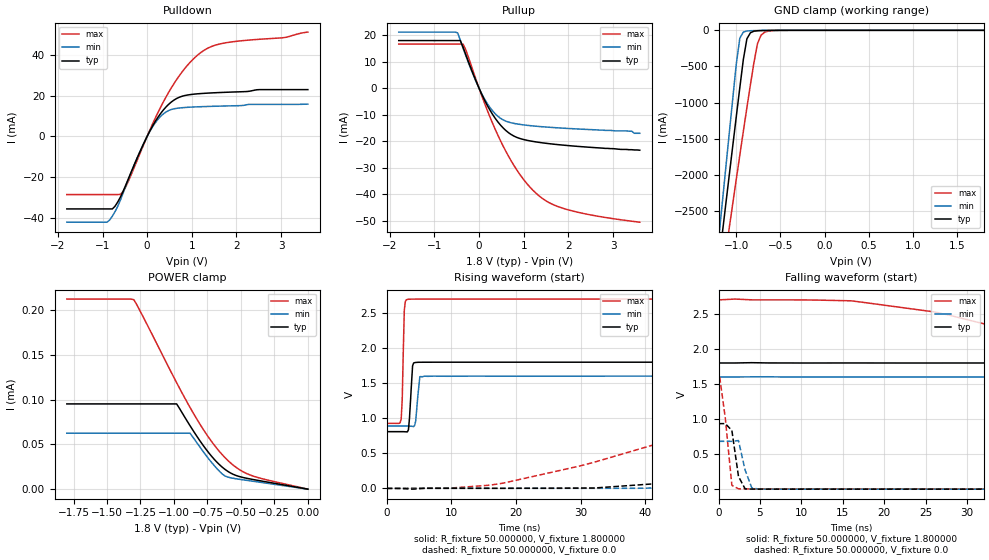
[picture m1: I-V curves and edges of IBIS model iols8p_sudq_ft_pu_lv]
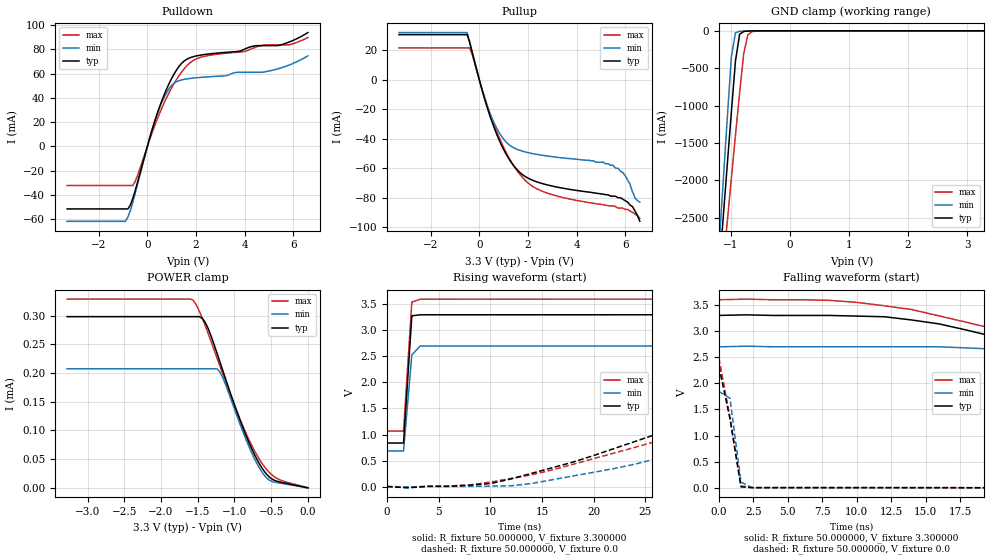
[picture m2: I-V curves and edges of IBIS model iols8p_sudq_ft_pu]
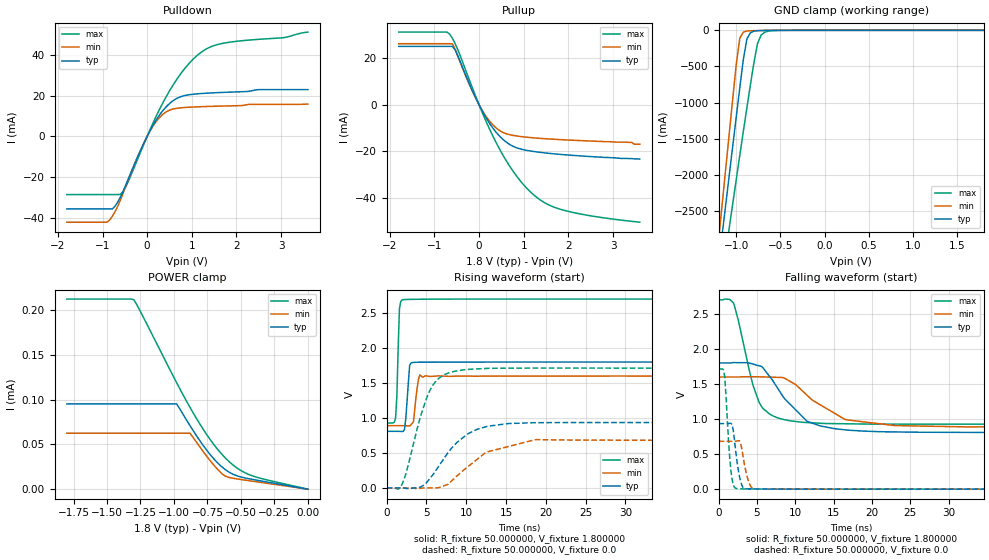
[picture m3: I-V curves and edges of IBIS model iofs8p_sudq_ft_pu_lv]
| IBIS file stm32wl33_vfqfpn32.ibs
[IBIS ver] 4.2
[File name] stm32wl33_vfqfpn32.ibs
[File Rev] 1.0
[Date]  24-06-2024
[Source] Data Created at STMicroelectronics
[Notes]  File originated from ELDO simulations.
[Disclaimer]  This information is for modeling purpose only and is
   not guaranteed. The information is subject to change without
   notice.
[Copyright] Copyright 2024 STMicroelectronics Inc.
|   Component stm32wl33_vfqfpn32
[Component] stm32wl33_vfqfpn32
[Manufacturer] STMicroelectronics
[Package]
| variable   typ   min   max
R_pkg  0  NA  NA
L_pkg  0  NA  NA
C_pkg  0  NA  NA
[Pin]   signal_name   model_name
1  PA2  io8prog2m25m50m120m_sudq_ft
2  PA3  io8prog2m25m50m120m_sudq_ft
3  VDD_1  power
4  PA0  io8prog2m25m50m120m_sudq_i2c_ft
5  PA11  io8prog2m25m50m120m_sudq_ft
6  PA10  io8prog2m25m50m120m_sudq_ft
7  PA9  io8prog2m25m50m120m_sudq_ft
8  PA8  io8prog2m25m50m120m_sudq_ft
9  PB6  io8prog2m25m50m120m_sudq_i2c_ft
10  PB12  io8prog2m25m50m120m_sudq_ft
11  PB13  io8prog2m25m50m120m_sudq_ft
12  PB14  io8prog2m25m50m120m_sudq_ft
13  PB15  io8prog2m25m50m120m_sudq_ft
14  LPAWUR  nc
15  RX  nc
16  EXTGND  gnd
17  TX_HP  nc
18  TX  nc
19  VDDRF  nc
20  OSCOUT  nc
21  OSCIN  nc
22  PA1  io8prog2m25m50m120m_sudq_i2c_ft
23  PB7  io8prog2m25m50m120m_sudq_i2c_ft
24  NRST  nc
25  VDDSD  nc
26  VLXSD  nc
27  VSSSD  nc
28  VFBSD  nc
29  VCAP  nc
30  PB0  io8prog2m25m50m120m_sudq_ft
31  PB1  io8prog2m25m50m120m_sudq_ft
32  PB2  io8prog2m25m50m120m_sudq_ft
0  EXTGND  gnd
[Package Model]   4l0-qfn-5x5-32-100mhz-230713
[Pin Mapping]   pulldown_ref   pullup_ref   | Comment
1  gndio  vddio
2  gndio  vddio
3  nc  vddio
4  gndio  vddio
5  gndio  vddio
6  gndio  vddio
7  gndio  vddio
8  gndio  vddio
9  gndio  vddio
10  gndio  vddio
11  gndio  vddio
12  gndio  vddio
13  gndio  vddio
14  nc  nc
15  nc  nc
16  gndio  nc
17  nc  nc
18  nc  nc
19  nc  nc
20  nc  nc
21  nc  nc
22  gndio  vddio
23  gndio  vddio
24  nc  nc
25  nc  nc
26  nc  nc
27  nc  nc
28  nc  nc
29  nc  nc
30  gndio  vddio
31  gndio  vddio
32  gndio  vddio
0  gndio  nc
[Model Selector] io8prog2m25m50m120m_sudq_ft
iols8p_sudq_ft_pd_lv  "IO low speed, PD=40kOhm - 1P8V"
iols8p_sudq_ft_pu_lv  "IO low speed, PU=40kOhm - 1P8V"
iols8p_sudq_ft_lv  "IO low speed - 1P8V"
iols8p_sudq_ft_pd  "IO low speed, PD=40kOhm - 3P3V"
iols8p_sudq_ft_pu  "IO low speed, PU=40kOhm - 3P3V"
iols8p_sudq_ft  "IO low speed - 3P3V"
iofs8p_sudq_ft_pd_lv  "IO full speed, PD=40kOhm - 1P8V"
iofs8p_sudq_ft_pu_lv  "IO full speed, PU=40kOhm - 1P8V"
iofs8p_sudq_ft_lv  "IO full speed - 1P8V"
iofs8p_sudq_ft_pd  "IO full speed, PD=40kOhm - 3P3V"
iofs8p_sudq_ft_pu  "IO full speed, PU=40kOhm - 3P3V"
iofs8p_sudq_ft  "IO full speed - 3P3V"
ioms8p_sudq_ft_pd_lv  "IO medium speed, PD=40kOhm - 1P8V"
ioms8p_sudq_ft_pu_lv  "IO medium speed, PU=40kOhm - 1P8V"
ioms8p_sudq_ft_lv  "IO medium speed - 1P8V"
ioms8p_sudq_ft_pd  "IO medium speed, PD=40kOhm - 3P3V"
ioms8p_sudq_ft_pu  "IO medium speed, PU=40kOhm - 3P3V"
ioms8p_sudq_ft  "IO medium speed - 3P3V"
iohs8p_sudq_ft_pd_lv  "IO high speed, PD=40kOhm - 1P8V"
iohs8p_sudq_ft_pu_lv  "IO high speed, PU=40kOhm - 1P8V"
iohs8p_sudq_ft_lv  "IO high speed - 1P8V"
iohs8p_sudq_ft_pd  "IO high speed, PD=40kOhm - 3P3V"
iohs8p_sudq_ft_pu  "IO high speed, PU=40kOhm - 3P3V"
iohs8p_sudq_ft  "IO high speed - 3P3V"
[Model Selector] io8prog2m25m50m120m_sudq_i2c_ft
iols8p_sudq_ft_pd_lv  "IO low speed, PD=40kOhm - 1P8V"
iols8p_sudq_ft_pu_lv  "IO low speed, PU=40kOhm - 1P8V"
iols8p_sudq_ft_lv  "IO low speed - 1P8V"
iols8p_sudq_ft_pd  "IO low speed, PD=40kOhm - 3P3V"
iols8p_sudq_ft_pu  "IO low speed, PU=40kOhm - 3P3V"
iols8p_sudq_ft  "IO low speed - 3P3V"
iofs8p_sudq_ft_pd_lv  "IO full speed, PD=40kOhm - 1P8V"
iofs8p_sudq_ft_pu_lv  "IO full speed, PU=40kOhm - 1P8V"
iofs8p_sudq_ft_lv  "IO full speed - 1P8V"
iofs8p_sudq_ft_pd  "IO full speed, PD=40kOhm - 3P3V"
iofs8p_sudq_ft_pu  "IO full speed, PU=40kOhm - 3P3V"
iofs8p_sudq_ft  "IO full speed - 3P3V"
ioms8p_sudq_ft_pd_lv  "IO medium speed, PD=40kOhm - 1P8V"
ioms8p_sudq_ft_pu_lv  "IO medium speed, PU=40kOhm - 1P8V"
ioms8p_sudq_ft_lv  "IO medium speed - 1P8V"
ioms8p_sudq_ft_pd  "IO medium speed, PD=40kOhm - 3P3V"
ioms8p_sudq_ft_pu  "IO medium speed, PU=40kOhm - 3P3V"
ioms8p_sudq_ft  "IO medium speed - 3P3V"
iohs8p_sudq_ft_pd_lv  "IO high speed, PD=40kOhm - 1P8V"
iohs8p_sudq_ft_pu_lv  "IO high speed, PU=40kOhm - 1P8V"
iohs8p_sudq_ft_lv  "IO high speed - 1P8V"
iohs8p_sudq_ft_pd  "IO high speed, PD=40kOhm - 3P3V"
iohs8p_sudq_ft_pu  "IO high speed, PU=40kOhm - 3P3V"
iohs8p_sudq_ft  "IO high speed - 3P3V"
io8_ft_i2c_ls_1v2   "GPIO I2C open-drain - 5V tolerant - 1.2V range - Low speed"
io8_ft_i2c_ms_1v2   "GPIO I2C open-drain - 5V tolerant - 1.2V range - Med speed"
io8_ft_i2c_fs_1v2   "GPIO I2C open-drain - 5V tolerant - 1.2V range - Fast speed"
io8_ft_i2c_hs_1v2   "GPIO I2C open-drain - 5V tolerant - 1.2V range - High speed"
io8_ft_i2c_ls_1v8   "GPIO I2C open-drain - 5V tolerant - 1.8V range - Low speed"
io8_ft_i2c_ms_1v8   "GPIO I2C open-drain - 5V tolerant - 1.8V range - Med speed"
io8_ft_i2c_fs_1v8   "GPIO I2C open-drain - 5V tolerant - 1.8V range - Fast speed"
io8_ft_i2c_hs_1v8   "GPIO I2C open-drain - 5V tolerant - 1.8V range - High speed"
io8_ft_i2c_ls_3v3   "GPIO I2C open-drain - 5V tolerant - 3.3V range - Low speed"
io8_ft_i2c_ms_3v3   "GPIO I2C open-drain - 5V tolerant - 3.3V range - Med speed"
io8_ft_i2c_fs_3v3   "GPIO I2C open-drain - 5V tolerant - 3.3V range - Fast speed"
io8_ft_i2c_hs_3v3   "GPIO I2C open-drain - 5V tolerant - 3.3V range - High speed"
io8_ft_i2c_fmp_3v3   "GPIO I2C open-drain fm+ - 5V tolerant - 3.3V range"
[Define Package Model]  4l0-qfn-5x5-32-100mhz-230713
[Manufacturer]  Unknown
[OEM]  Unknown
[Description]  None
[Number Of Pins]  32
[Pin Numbers]
| Pin Num   Terminal Name
14 | LPAWUR
4 | PA0
22 | PA1
1 | PA2
2 | PA3
8 | PA8
7 | PA9
6 | PA10
5 | PA11
30 | PB0
31 | PB1
32 | PB2
9 | PB6
23 | PB7
10 | PB12
11 | PB13
12 | PB14
13 | PB15
21 | OSCIN
20 | OSCOUT
27 | VSSSD
24 | NRST
15 | RX
28 | VFBSD
26 | VLXSD
18 | TX
17 | TX_HP
19 | VDDRF
3 | VDD_1
29 | VCAP
25 | VDDSD
16 | EXTGND
[Model Data]
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[End Model Data]
[End Package Model]
| Models and submodels in the file (37): iols8p_sudq_ft_pd_lv (I/O), iols8p_sudq_ft_pu_lv (I/O), iols8p_sudq_ft_lv (I/O), iols8p_sudq_ft_pd (I/O), iols8p_sudq_ft_pu (I/O), iols8p_sudq_ft (I/O), iofs8p_sudq_ft_pd_lv (I/O), iofs8p_sudq_ft_pu_lv (I/O), iofs8p_sudq_ft_lv (I/O), iofs8p_sudq_ft_pd (I/O), iofs8p_sudq_ft_pu (I/O), iofs8p_sudq_ft (I/O), ioms8p_sudq_ft_pd_lv (I/O), ioms8p_sudq_ft_pu_lv (I/O), ioms8p_sudq_ft_lv (I/O), ioms8p_sudq_ft_pd (I/O), ioms8p_sudq_ft_pu (I/O), ioms8p_sudq_ft (I/O), iohs8p_sudq_ft_pd_lv (I/O), iohs8p_sudq_ft_pu_lv (I/O), iohs8p_sudq_ft_lv (I/O), iohs8p_sudq_ft_pd (I/O), iohs8p_sudq_ft_pu (I/O), iohs8p_sudq_ft (I/O), io8_ft_i2c_fs_1v2 (I/O_open_drain), io8_ft_i2c_hs_1v2 (I/O_open_drain), io8_ft_i2c_ls_1v2 (I/O_open_drain), io8_ft_i2c_ms_1v2 (I/O_open_drain), io8_ft_i2c_fs_1v8 (I/O_open_drain), io8_ft_i2c_hs_1v8 (I/O_open_drain), io8_ft_i2c_ls_1v8 (I/O_open_drain), io8_ft_i2c_ms_1v8 (I/O_open_drain), io8_ft_i2c_fs_3v3 (I/O_open_drain), io8_ft_i2c_hs_3v3 (I/O_open_drain), io8_ft_i2c_ls_3v3 (I/O_open_drain), io8_ft_i2c_ms_3v3 (I/O_open_drain), io8_ft_i2c_fmp_3v3 (I/O_open_drain)
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|   Model iols8p_sudq_ft_pu_lv
[Model]  iols8p_sudq_ft_pu_lv
Model_type I/O
Polarity   Non-Inverting
Enable   Active-Low
Vinl =   0.540000V
Vinh =   1.260000V
Vmeas =  0.900000V
Cref =   50.000000pF
Rref =   100.000000M
Vref =   0.0V
C_comp   1.984800pF   1.899400pF   2.077500pF
[Temperature Range]   25.000000   -40.000000   0.125000k
[Pullup Reference]   1.800000V   1.600000V   2.700000V
[Pulldown Reference]   0.0V   0.0V   0.0V
[POWER Clamp Reference]   1.800000V   1.600000V   2.700000V
[GND Clamp Reference]   0.0V   0.0V   0.0V
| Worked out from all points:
|   slope of the pulldown table from 0 to 0.27 V, typ, clamps not added: 26.4 ohm
|   slope of the pullup table from 0 to 0.27 V, typ, clamps not added: 30.1 ohm
|   GND clamp passes 1 mA (typ) near -0.61 V on its own axis
|   rising waveform, R_fixture 50.000000, V_fixture 1.800000: 20-80 % time 379ps typ, 423ps min, 265ps max; typ from 0.81 V to 1.8 V
|   rising waveform, R_fixture 50.000000, V_fixture 0.0: 20-80 % time 68.6ns typ, 74.3ns min, 45.2ns max; typ from 0.001 V to 0.935 V
|   falling waveform, R_fixture 50.000000, V_fixture 1.800000: 20-80 % time 72.7ns typ, 95.3ns min, 37.6ns max; typ from 1.8 V to 0.81 V
|   falling waveform, R_fixture 50.000000, V_fixture 0.0: 20-80 % time 683ps typ, 950ps min, 966ps max; typ from 0.935 V to 0.001 V
[Pulldown]
|Voltage   I(typ)   I(min)   I(max)
-1.8V     -35.64mA   -42.15mA   -28.59mA
-900mV    -35.64mA   -42.15mA   -28.59mA
-780mV    -35.64mA   -39.2mA    -28.59mA
-600mV    -29.83mA   -31.3mA    -28.52mA
-420mV    -20.8mA    -21.07mA   -21.98mA
60mV      2.604mA    2.459mA    3.062mA
240mV     9.303mA    8.31mA     11.61mA
480mV     15.67mA    12.64mA    21.52mA
720mV     19.18mA    13.9mA     29.74mA
960mV     20.46mA    14.3mA     36.27mA
1.44V     21.29mA    14.7mA     44.06mA
3.6V      22.91mA    15.79mA    51.15mA
[Pullup]
|Voltage   I(typ)   I(min)   I(max)
-1.8V     18.05mA    21.25mA    16.71mA
-540mV    18.05mA    21.25mA    16.71mA
-480mV    18.05mA    20.96mA    16.71mA
-420mV    18.05mA    18.11mA    16.71mA
-360mV    15.57mA    15.21mA    16.71mA
60mV      -2.268mA   -2.095mA   -2.822mA
360mV     -11.31mA   -9.605mA   -15.45mA
600mV     -15.96mA   -12.42mA   -23.82mA
840mV     -18.52mA   -13.44mA   -30.72mA
1.38V     -20.52mA   -14.48mA   -41.14mA
2.1V      -21.8mA    -15.27mA   -46.39mA
3.6V      -23.4mA    -17mA      -50.6mA
[GND_clamp]
|Voltage   I(typ)   I(min)   I(max)
-1.8V     -9.477A    -9.805A    -9.016A
-1.2V     -3.243A    -2.9A      -3.759A
-1.16V    -2.83A     -2.409A    -3.417A
-1.12V    -2.418A    -1.919A    -3.076A
-1.08V    -2.008A    -1.431A    -2.736A
-1V       -1.194A    -466mA     -2.061A
-960mV    -792.8mA   -108.7mA   -1.727A
-920mV    -402mA     -24.35mA   -1.396A
-880mV    -117.8mA   -9.188mA   -1.071A
-760mV    -5.896mA   -2.88mA    -183.8mA
-680mV    -2.395mA   -1.099mA   -26.61mA
1.8V      0A         0A         0A
[POWER_clamp]
|Voltage   I(typ)   I(min)   I(max)
-1.8V     95.27uA    62.52uA    212.4uA
-1.3V     95.27uA    62.52uA    211.7uA
-1.24V    95.27uA    62.52uA    195.4uA
-980mV    95.27uA    62.52uA    119uA
-880mV    70.93uA    62.52uA    91.35uA
-740mV    40.61uA    33.79uA    57.65uA
-640mV    24.64uA    16.99uA    38.63uA
-600mV    20.11uA    13.6uA     32.43uA
-540mV    15.51uA    11.72uA    24.8uA
-440mV    11.66uA    9.491uA    16.35uA
-340mV    8.934uA    7.326uA    11.65uA
0V        0A         0A         0A
[Ramp]
| variable   typ   min   max
dV/dt_r  0.56095/68.67975n   0.40953/74.27229n   1.02717/44.98407n
dV/dt_f  0.59405/72.60739n   0.42589/95.26095n   1.06315/37.53994n
R_load = 50.000000
[Rising Waveform]
R_fixture= 50.000000
V_fixture= 1.800000
V_fixture_min= 1.600000
V_fixture_max= 2.700000
|time   V(typ)   V(min)   V(max)
0s        809.8mV    890.3mV    928.1mV
2.242ns   809.8mV    890.3mV    993.3mV
2.402ns   809.8mV    890.3mV    1.271V
2.723ns   809mV      890.3mV    2.541V
3.203ns   807.2mV    890.4mV    2.695V
4.004ns   1.748V     884.3mV    2.699V
4.484ns   1.796V     960.8mV    2.699V
5.125ns   1.799V     1.593V     2.7V
5.766ns   1.8V       1.6V       2.7V
79.76ns   1.8V       1.6V       2.7V
[Rising Waveform]
R_fixture= 50.000000
V_fixture= 0.0
V_fixture_min= 0.0
V_fixture_max= 0.0
|time   V(typ)   V(min)   V(max)
0s        727.8uV    547uV      1.255mV
18.02ns   2.02mV     1.674mV    75.77mV
32.03ns   6.18mV     1.697mV    372.5mV
62.06ns   209.3mV    74.21mV    1.129V
80.08ns   398.5mV    158mV      1.429V
104.1ns   610.5mV    330.5mV    1.601V
126.1ns   738.8mV    448.3mV    1.661V
174.2ns   885.5mV    630.8mV    1.704V
248.2ns   930.2mV    683.3mV    1.714V
997ns     935.3mV    683.1mV    1.714V
[Falling Waveform]
R_fixture= 50.000000
V_fixture= 1.800000
V_fixture_min= 1.600000
V_fixture_max= 2.700000
|time   V(typ)   V(min)   V(max)
0s        1.8V       1.6V       2.7V
16.02ns   1.8V       1.6V       2.687V
26.03ns   1.8V       1.6V       2.529V
64.06ns   1.737V     1.6V       1.391V
76.08ns   1.647V     1.6V       1.186V
120.1ns   1.255V     1.504V     992.1mV
160.2ns   977.5mV    1.286V     953.6mV
200.2ns   882.5mV    1.065V     936.8mV
314.3ns   819.5mV    908.5mV    928.2mV
997ns     809.8mV    890.3mV    928.1mV
[Falling Waveform]
R_fixture= 50.000000
V_fixture= 0.0
V_fixture_min= 0.0
V_fixture_max= 0.0
|time   V(typ)   V(min)   V(max)
0s        935.3mV    683.1mV    1.714V
800.8ps   935.3mV    683.1mV    1.021V
1.602ns   838.7mV    682.5mV    55.24mV
2.402ns   181.5mV    693.4mV    5.324mV
3.203ns   4.882mV    272.1mV    4.519mV
4.004ns   1.823mV    19.9mV     4.432mV
4.805ns   1.435mV    1.988mV    4.408mV
79.28ns   727.8uV    547uV      1.255mV
|   Model iols8p_sudq_ft_pu
[Model]  iols8p_sudq_ft_pu
Model_type I/O
Polarity   Non-Inverting
Enable   Active-Low
Vinl =   0.990000V
Vinh =   2.310000V
Vmeas =  1.650000V
Cref =   50.000000pF
Rref =   100.000000M
Vref =   0.0V
C_comp   2.036400pF   1.984000pF   2.082300pF
[Temperature Range]   25.000000   -40.000000   0.125000k
[Pullup Reference]   3.300000V   2.700000V   3.600000V
[Pulldown Reference]   0.0V   0.0V   0.0V
[POWER Clamp Reference]   3.300000V   2.700000V   3.600000V
[GND Clamp Reference]   0.0V   0.0V   0.0V
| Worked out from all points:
|   slope of the pulldown table from 0 to 0.495 V, typ, clamps not added: 15.4 ohm
|   slope of the pullup table from 0 to 0.495 V, typ, clamps not added: 18.1 ohm
|   GND clamp passes 1 mA (typ) near -0.60 V on its own axis
|   rising waveform, R_fixture 50.000000, V_fixture 3.300000: 20-80 % time 485ps typ, 525ps min, 492ps max; typ from 0.836 V to 3.3 V
|   rising waveform, R_fixture 50.000000, V_fixture 0.0: 20-80 % time 24.4ns typ, 26.2ns min, 30.7ns max; typ from 0.001 V to 2.33 V
|   falling waveform, R_fixture 50.000000, V_fixture 3.300000: 20-80 % time 21.2ns typ, 25.4ns min, 23.9ns max; typ from 3.3 V to 0.836 V
|   falling waveform, R_fixture 50.000000, V_fixture 0.0: 20-80 % time 956ps typ, 552ps min, 969ps max; typ from 2.33 V to 0.001 V
[Pulldown]
|Voltage   I(typ)   I(min)   I(max)
-3.3V     -51.62mA   -61.84mA   -32.32mA
-900mV    -51.62mA   -61.84mA   -32.32mA
-800mV    -51.62mA   -58.24mA   -32.32mA
-500mV    -36.51mA   -38.7mA    -28.96mA
400mV     26.66mA    26.58mA    22.18mA
800mV     47.72mA    44.74mA    40.6mA
1.1V      59.79mA    52.18mA    51.93mA
1.5V      70.22mA    55.24mA    63.66mA
2.1V      74.97mA    56.75mA    72.88mA
4.9V      83.13mA    61.75mA    83.74mA
5.8V      85.85mA    66.87mA    83.74mA
6.6V      93.9mA     74.68mA    89.84mA
[Pullup]
|Voltage   I(typ)   I(min)   I(max)
-3.3V     30.51mA    31.92mA    21.54mA
-500mV    30.51mA    31.92mA    21.54mA
-300mV    19.24mA    18.93mA    17.46mA
500mV     -27.53mA   -25.31mA   -25.83mA
1V        -47.29mA   -40.29mA   -45.86mA
1.5V      -60.05mA   -46.83mA   -60.43mA
2V        -66.7mA    -49.43mA   -69.91mA
2.7V      -70.92mA   -51.53mA   -76.32mA
5.5V      -79mA      -58mA      -85.6mA
6V        -82mA      -65mA      -88mA
6.3V      -86mA      -76mA      -90mA
6.6V      -96mA      -83mA      -94mA
[GND_clamp]
|Voltage   I(typ)   I(min)   I(max)
-3.3V     -9.812A    -9.822A    -9.937A
-1.2V     -3.251A    -2.905A    -3.763A
-1.13V    -2.527A    -2.046A    -3.165A
-1.06V    -1.808A    -1.191A    -2.57A
-990mV    -1.097A    -352.6mA   -1.979A
-920mV    -404.2mA   -25.08mA   -1.398A
-850mV    -46.53mA   -6.503mA   -832.3mA
-780mV    -8.496mA   -3.578mA   -302.4mA
-710mV    -3.383mA   -1.716mA   -53.8mA
-640mV    -1.589mA   -553.8uA   -11.72mA
-360mV    -2.023uA   0A         -84.67uA
3.28V     0A         0A         0A
[POWER_clamp]
|Voltage   I(typ)   I(min)   I(max)
-3.28V    298.2uA    207.4uA    328.7uA
-1.56V    298.2uA    207.4uA    326.5uA
-1.48V    298.2uA    207.4uA    308.2uA
-1.4V     288.5uA    207.4uA    283.1uA
-1.24V    235.4uA    207.4uA    226.9uA
-1.2V     220.1uA    202.1uA    212.7uA
-1.12V    189.4uA    179.6uA    184.4uA
-920mV    116.5uA    109.4uA    118.1uA
-680mV    46.31uA    39.06uA    53.8uA
-560mV    23.38uA    16.91uA    31.65uA
-480mV    14.66uA    10.76uA    21.51uA
0V        0A         0A         0A
[Ramp]
| variable   typ   min   max
dV/dt_r  1.39432/24.32907n   1.10712/26.03302n   1.49022/30.66754n
dV/dt_f  1.47837/21.11983n   1.20959/25.32351n   1.52028/23.79583n
R_load = 50.000000
[Rising Waveform]
R_fixture= 50.000000
V_fixture= 3.300000
V_fixture_min= 2.700000
V_fixture_max= 3.600000
|time   V(typ)   V(min)   V(max)
0s        836mV      684mV      1.066V
1.602ns   835.8mV    683.5mV    1.067V
2.402ns   3.279V     2.529V     3.543V
3.203ns   3.299V     2.699V     3.598V
79.28ns   3.3V       2.7V       3.6V
[Rising Waveform]
R_fixture= 50.000000
V_fixture= 0.0
V_fixture_min= 0.0
V_fixture_max= 0.0
|time   V(typ)   V(min)   V(max)
0s        932.5uV    605.4uV    1.507mV
10.01ns   58.21mV    9.253mV    85.87mV
14.01ns   255mV      59.61mV    227.5mV
22.02ns   733mV      347.4mV    646.1mV
34.03ns   1.487V     931.9mV    1.309V
46.05ns   1.978V     1.401V     1.857V
58.06ns   2.166V     1.659V     2.17V
86.09ns   2.285V     1.807V     2.399V
188.2ns   2.326V     1.846V     2.486V
997ns     2.325V     1.846V     2.486V
[Falling Waveform]
R_fixture= 50.000000
V_fixture= 3.300000
V_fixture_min= 2.700000
V_fixture_max= 3.600000
|time   V(typ)   V(min)   V(max)
0s        3.3V       2.7V       3.6V
8.008ns   3.3V       2.7V       3.589V
16.02ns   3.136V     2.699V     3.289V
24.02ns   2.583V     2.575V     2.745V
38.04ns   1.562V     1.936V     1.818V
46.05ns   1.184V     1.512V     1.461V
54.05ns   1.038V     1.14V      1.302V
62.06ns   969.1mV    930.8mV    1.229V
88.09ns   885.8mV    756.3mV    1.123V
997ns     836mV      684mV      1.066V
[Falling Waveform]
R_fixture= 50.000000
V_fixture= 0.0
V_fixture_min= 0.0
V_fixture_max= 0.0
|time   V(typ)   V(min)   V(max)
0s        2.325V     1.846V     2.486V
800.8ps   1.327V     1.716V     1.355V
1.602ns   20.24mV    111mV      36.22mV
2.402ns   4.804mV    3.818mV    6.652mV
79.28ns   932.5uV    605.4uV    1.507mV
|   Model iofs8p_sudq_ft_pu_lv
[Model]  iofs8p_sudq_ft_pu_lv
Model_type I/O
Polarity   Non-Inverting
Enable   Active-Low
Vinl =   0.540000V
Vinh =   1.260000V
Vmeas =  0.900000V
Cref =   40.000000pF
Rref =   100.000000M
Vref =   0.0V
C_comp   1.984800pF   1.899400pF   2.077500pF
[Temperature Range]   25.000000   -40.000000   0.125000k
[Pullup Reference]   1.800000V   1.600000V   2.700000V
[Pulldown Reference]   0.0V   0.0V   0.0V
[POWER Clamp Reference]   1.800000V   1.600000V   2.700000V
[GND Clamp Reference]   0.0V   0.0V   0.0V
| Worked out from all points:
|   slope of the pulldown table from 0 to 0.27 V, typ, clamps not added: 26.4 ohm
|   slope of the pullup table from 0 to 0.27 V, typ, clamps not added: 30.1 ohm
|   GND clamp passes 1 mA (typ) near -0.61 V on its own axis
|   rising waveform, R_fixture 50.000000, V_fixture 1.800000: 20-80 % time 376ps typ, 425ps min, 278ps max; typ from 0.81 V to 1.8 V
|   rising waveform, R_fixture 50.000000, V_fixture 0.0: 20-80 % time 4.11ns typ, 5.19ns min, 2.6ns max; typ from 0.001 V to 0.935 V
|   falling waveform, R_fixture 50.000000, V_fixture 1.800000: 20-80 % time 4.49ns typ, 5.53ns min, 2.44ns max; typ from 1.8 V to 0.81 V
|   falling waveform, R_fixture 50.000000, V_fixture 0.0: 20-80 % time 698ps typ, 764ps min, 598ps max; typ from 0.935 V to 0.001 V
[Pulldown]
|Voltage   I(typ)   I(min)   I(max)
-1.8V     -35.64mA   -42.15mA   -28.59mA
-900mV    -35.64mA   -42.15mA   -28.59mA
-780mV    -35.64mA   -39.2mA    -28.59mA
-600mV    -29.83mA   -31.3mA    -28.52mA
-420mV    -20.8mA    -21.07mA   -21.98mA
60mV      2.604mA    2.459mA    3.062mA
240mV     9.303mA    8.31mA     11.61mA
480mV     15.67mA    12.64mA    21.52mA
720mV     19.18mA    13.9mA     29.74mA
960mV     20.46mA    14.3mA     36.27mA
1.44V     21.29mA    14.7mA     44.06mA
3.6V      22.91mA    15.79mA    51.15mA
[Pullup]
|Voltage   I(typ)   I(min)   I(max)
-1.8V     25.2mA     26.34mA    31.35mA
-660mV    25.2mA     26.34mA    30.46mA
-600mV    25.2mA     26.34mA    28.76mA
-540mV    23.79mA    24.11mA    26.53mA
-60mV     2.392mA    2.26mA     2.893mA
300mV     -9.801mA   -8.48mA    -13.12mA
480mV     -13.91mA   -11.33mA   -19.82mA
720mV     -17.48mA   -13.04mA   -27.45mA
1.26V     -20.22mA   -14.3mA    -39.41mA
1.56V     -20.91mA   -14.71mA   -43.13mA
1.98V     -21.62mA   -15.16mA   -45.85mA
3.6V      -23.4mA    -17mA      -50.6mA
[GND_clamp]
|Voltage   I(typ)   I(min)   I(max)
-1.8V     -9.477A    -9.805A    -9.016A
-1.2V     -3.243A    -2.9A      -3.759A
-1.16V    -2.83A     -2.409A    -3.417A
-1.12V    -2.418A    -1.919A    -3.076A
-1.08V    -2.008A    -1.431A    -2.736A
-1V       -1.194A    -466mA     -2.061A
-960mV    -792.8mA   -108.7mA   -1.727A
-920mV    -402mA     -24.35mA   -1.396A
-880mV    -117.8mA   -9.188mA   -1.071A
-760mV    -5.896mA   -2.88mA    -183.8mA
-680mV    -2.395mA   -1.099mA   -26.61mA
1.8V      0A         0A         0A
[POWER_clamp]
|Voltage   I(typ)   I(min)   I(max)
-1.8V     95.27uA    62.52uA    212.4uA
-1.3V     95.27uA    62.52uA    211.7uA
-1.24V    95.27uA    62.52uA    195.4uA
-980mV    95.27uA    62.52uA    119uA
-880mV    70.93uA    62.52uA    91.35uA
-740mV    40.61uA    33.79uA    57.65uA
-640mV    24.64uA    16.99uA    38.63uA
-600mV    20.11uA    13.6uA     32.43uA
-540mV    15.51uA    11.72uA    24.8uA
-440mV    11.66uA    9.491uA    16.35uA
-340mV    8.934uA    7.326uA    11.65uA
0V        0A         0A         0A
[Ramp]
| variable   typ   min   max
dV/dt_r  0.56065/4.10666n   0.41004/5.21865n   1.02723/2.59603n
dV/dt_f  0.59442/4.48383n   0.42528/5.51382n   1.06315/2.43914n
R_load = 50.000000
[Rising Waveform]
R_fixture= 50.000000
V_fixture= 1.800000
V_fixture_min= 1.600000
V_fixture_max= 2.700000
|time   V(typ)   V(min)   V(max)
0s        809.8mV    890.3mV    928.1mV
1.121ns   809.8mV    890.3mV    1.004V
1.281ns   809.8mV    890.3mV    1.323V
1.602ns   809.1mV    890.3mV    2.561V
2.082ns   807.7mV    890.4mV    2.691V
2.402ns   997mV      889.9mV    2.694V
2.883ns   1.749V     885.5mV    2.696V
3.363ns   1.794V     947.3mV    2.697V
4.164ns   1.798V     1.617V     2.698V
79.76ns   1.8V       1.6V       2.7V
[Rising Waveform]
R_fixture= 50.000000
V_fixture= 0.0
V_fixture_min= 0.0
V_fixture_max= 0.0
|time   V(typ)   V(min)   V(max)
0s        728.8uV    547.7uV    1.257mV
1.441ns   744.3uV    546.4uV    -16.91mV
2.082ns   506uV      547.1uV    92.43mV
4.324ns   19.48mV    -2.981mV   1.051V
5.766ns   182.9mV    1.182mV    1.462V
8.488ns   610.6mV    135.8mV    1.667V
10.25ns   777mV      308.1mV    1.695V
12.49ns   876.1mV    511.9mV    1.708V
18.74ns   932.8mV    690.8mV    1.714V
79.76ns   935.3mV    683.1mV    1.713V
[Falling Waveform]
R_fixture= 50.000000
V_fixture= 1.800000
V_fixture_min= 1.600000
V_fixture_max= 2.700000
|time   V(typ)   V(min)   V(max)
0s        1.8V       1.6V       2.7V
1.922ns   1.806V     1.6V       2.659V
4.484ns   1.785V     1.604V     1.484V
5.285ns   1.76V      1.603V     1.239V
8.649ns   1.287V     1.58V      989.9mV
11.53ns   969.5mV    1.341V     950.8mV
13.29ns   901.2mV    1.201V     940.5mV
16.66ns   844.7mV    990mV      932.8mV
22.9ns    817.1mV    908.3mV    928.2mV
79.76ns   809.8mV    890.3mV    928.1mV
[Falling Waveform]
R_fixture= 50.000000
V_fixture= 0.0
V_fixture_min= 0.0
V_fixture_max= 0.0
|time   V(typ)   V(min)   V(max)
0s        935.3mV    683.1mV    1.713V
800.8ps   935.2mV    683.1mV    1.598V
1.602ns   939.6mV    683mV      265.7mV
1.922ns   835.1mV    682.6mV    56.69mV
2.402ns   395.6mV    688mV      8.372mV
2.883ns   109.8mV    649.6mV    4.938mV
3.203ns   20.99mV    464.8mV    4.14mV
4.004ns   4.338mV    82.51mV    3.072mV
4.645ns   3.697mV    5.197mV    2.535mV
79.76ns   728.8uV    547.7uV    1.257mV
